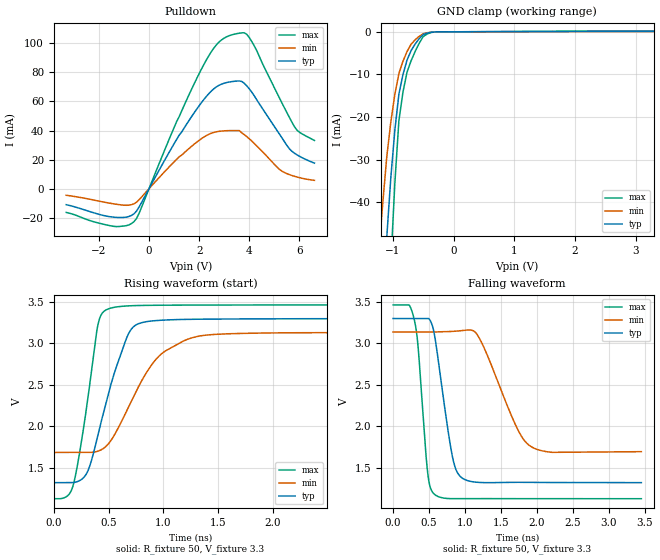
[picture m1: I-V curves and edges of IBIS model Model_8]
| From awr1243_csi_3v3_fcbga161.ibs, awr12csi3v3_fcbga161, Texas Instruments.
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| Model based on original model for BC1833DV40DCPBFBP18LL_OD_FS_SSDLV
|   Sub model BC40D_V_PD_ON_5P_!SC1_3P3
[model]   Model_8
|[Description]  [3.3V-I/O_OPEN_DRAIN-WEAK_PD_ON-FAST, IND, 5%]
|   FAST,WEAK_PD_ON,IND,5%
|[Input Load]   WEAK_PD_ON
|[Output Drive] FAST
|Voltage   3.3V
|Mode   I/O_OPEN_DRAIN
Model_type   I/O_open_drain
Polarity   Non-Inverting
Enable   Active-Low
Vinl =  0.8V
Vinh =  2V
Cref =  15pF
Rref =  100.0000M
Vref =  0V
Vmeas =  1.65
C_comp   2.059994p   1.862014p   2.067327p
[Model Spec]
Vinl   0.8V   0.8V   0.8V
Vinh   2V   2V   2V
[Temperature Range]   25   125   -40
[Voltage Range]   3.3   3.135   3.465
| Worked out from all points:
|   slope of the pulldown table from 0 to 0.495 V, typ, clamps not added: 31.8 ohm
|   GND clamp passes 1 mA (typ) near -0.52 V on its own axis
|   rising waveform, R_fixture 50, V_fixture 3.3: 20-80 % time 251ps typ, 371ps min, 151ps max; typ from 1.32 V to 3.3 V
|   falling waveform, R_fixture 50, V_fixture 3.3: 20-80 % time 196ps typ, 407ps min, 120ps max; typ from 3.3 V to 1.32 V
[Pulldown]
-3.3V     -10.92mA   -4.469mA   -16.24mA
-1.4V     -19.52mA   -10.37mA   -25.81mA
-600mV    -17.22mA   -10.34mA   -22.6mA
-400mV    -12.67mA   -7.623mA   -17.05mA
1.2V      36.7mA     21.92mA    49.35mA
2.1V      59.3mA     34.49mA    82.4mA
2.7V      70.09mA    39.15mA    99.03mA
3.3V      73.56mA    39.95mA    105.7mA
3.9V      70.66mA    35.84mA    106mA
5.2V      37.64mA    13.39mA    62.46mA
5.8V      24.43mA    8.578mA    42.66mA
6.6V      17.6mA     5.765mA    33.17mA
[GND_clamp]
-3.3V     -787.2mA   -627.7mA   -1.235A
-1.233V   -85.66mA   -52.14mA   -138.8mA
-1.167V   -66.47mA   -40.37mA   -107.7mA
-1.1V     -48.25mA   -29.37mA   -77.98mA
-1.033V   -34.28mA   -21.19mA   -54.56mA
-966.7mV  -23.07mA   -14.67mA   -35.51mA
-900mV    -14.62mA   -9.792mA   -20.84mA
-833.3mV  -10.07mA   -6.939mA   -14.17mA
-700mV    -4.435mA   -2.94mA    -6.836mA
-500mV    -641.2uA   -454.9uA   -1.12mA
-300mV    -31.62uA   -32.88uA   -44.11uA
3.3V      108.6uA    60.68uA    188uA
[Ramp]
dV/dt_f  1.1955351/0.19759568n 0.88985276/0.4200075n  1.4066392/0.12028585n
dV/dt_r  1.1906978/0.23429938n 0.88860778/0.46756332n  1.4192328/0.14138141n
R_load = 50
[Rising Waveform]
R_fixture = 50
V_fixture = 3.3
V_fixture_min = 3.135
V_fixture_max = 3.465
0s        1.321V     1.685V     1.128V
178.2ps   1.322V     1.685V     1.295V
301.2ps   1.435V     1.685V     2.241V
400ps     1.877V     1.699V     3.202V
481.7ps   2.307V     1.764V     3.404V
656.6ps   3.033V     2.161V     3.449V
724.7ps   3.194V     2.347V     3.453V
946.4ps   3.274V     2.825V     3.458V
1.232ns   3.288V     3.053V     3.46V
3.453ns   3.297V     3.129V     3.462V
[Falling Waveform]
R_fixture = 50
V_fixture = 3.3
V_fixture_min = 3.135
V_fixture_max = 3.465
0s        3.297V     3.134V     3.461V
297.1ps   3.297V     3.134V     3.274V
347.5ps   3.297V     3.134V     2.957V
481.9ps   3.297V     3.134V     1.432V
580.8ps   3.074V     3.135V     1.176V
820.1ps   1.656V     3.142V     1.128V
962.4ps   1.375V     3.152V     1.128V
1.188ns   1.324V     3.078V     1.129V
1.913ns   1.324V     1.758V     1.127V
3.453ns   1.321V     1.694V     1.127V
